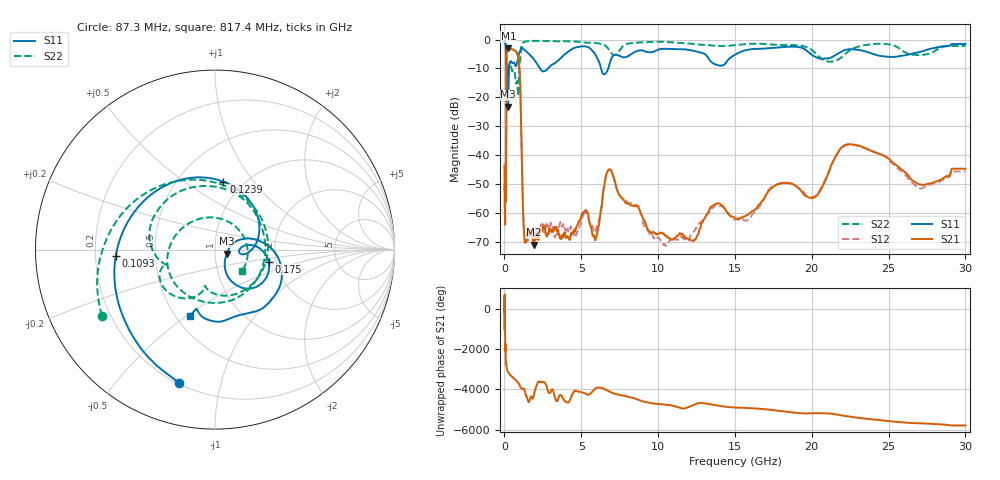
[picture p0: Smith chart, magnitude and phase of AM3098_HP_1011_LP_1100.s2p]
! Date/Time: Thu, Feb 28, 2019 8:43 AM
! Network Analyzer: Agilent Technologies E8364B Rev: A.07.50.67
! Sweep from 0.010 to 30.000 GHz, 1601 Points, Sweep Type: LOG
! Power Supply: 5.022 V, 0.002 A
# Hz S DB R 50
!freq MagS11 AngS11 MagS21 AngS21 MagS12 AngS12 MagS22 AngS22
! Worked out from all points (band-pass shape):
!   1601 points, 10 MHz to 30 GHz, reference 50 ohm
!   highest |S21| = -3.11 dB at 262.5 MHz (marker M1); lowest = -71.0 dB at 1.895 GHz (marker M2)
!   |S21| within 3 dB of the highest: 137.5 MHz to 887.5 MHz (750 MHz wide, 146 % of centre)
!   lowest |S11| = -23.2 dB at 242.3 MHz (marker M3), VSWR 1.15, Z = 56.9 - j2.63 ohm
!   |S11| at or under -10 dB: 192.5 MHz to 304.1 MHz (111.7 MHz wide, 45 % of centre); 2.321 GHz to 2.839 GHz (517.7 MHz wide, 20.1 % of centre); 6.283 GHz to 6.758 GHz (475.3 MHz wide, 7.29 % of centre)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
!   |S22| runs from -19.5 to -0.5 dB; largest |S21 - S12| = 0.012
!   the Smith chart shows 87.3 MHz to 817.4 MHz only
!   S11 on the Smith chart (normalised r, x): 87.3 MHz: 0.21, -0.74; 109.3 MHz: 0.29, -0.03; 123.9 MHz: 0.81, +0.72; 175 MHz: 1.83, -0.27; 817.4 MHz: 0.59, -0.51
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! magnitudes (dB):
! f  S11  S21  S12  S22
! 10 MHz  -0.3  -44.1  -43.3  -0.6
! 38.04 MHz  -0.4  -59.2  -62.7  -0.9
! 87.3 MHz  -2.3  -54.4  -55.0  -2.7
! 109.3 MHz  -5.1  -34.2  -34.1  -6.4
! 123.9 MHz  -8.4  -13.5  -13.5  -10.6
! 144.7 MHz  -17.2  -5.0  -5.0  -13.6
! 175 MHz  -10.3  -3.9  -3.9  -9.4
! 242.3 MHz  -23.2  -3.1  -3.1  -11.0
! 262.5 MHz  -17.0  -3.1  -3.1  -10.5
! 550.5 MHz  -8.1  -3.5  -3.5  -10.7
! 817.4 MHz  -8.1  -4.8  -4.8  -14.4
! 1.009 GHz  -4.1  -13.0  -13.0  -7.6
! 1.289 GHz  -3.6  -68.5  -66.0  -0.8
! 1.895 GHz  -6.7  -71.0  -69.1  -0.5
! 2.084 GHz  -8.1  -68.2  -66.0  -0.5
! 5.9 GHz  -5.0  -69.6  -66.8  -1.2
! 6.821 GHz  -8.8  -45.1  -45.0  -3.7
! 7.926 GHz  -6.0  -56.8  -55.8  -1.6
! 10.59 GHz  -3.2  -68.5  -70.8  -0.9
! 20.1 GHz  -5.6  -54.8  -54.5  -4.1
! 22.56 GHz  -3.4  -36.3  -36.5  -3.5
! 30 GHz  -1.6  -44.8  -45.7  -2.2
